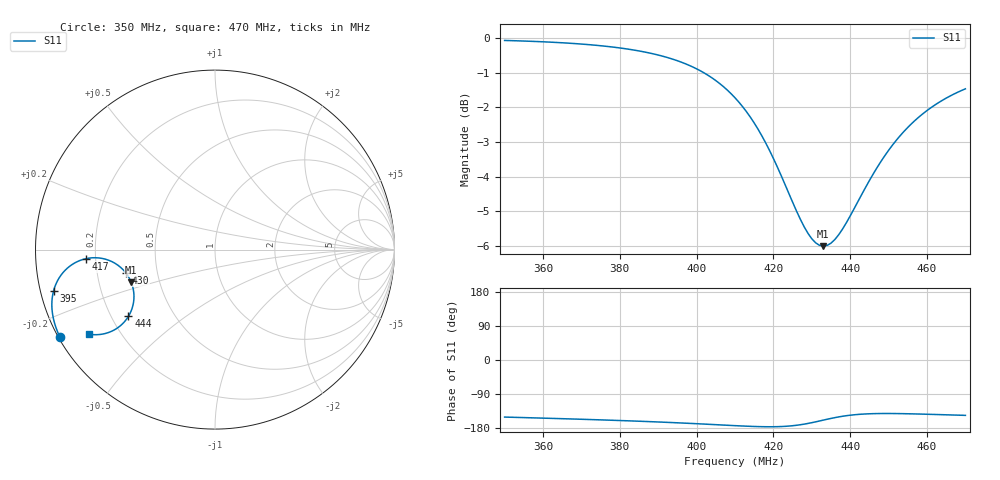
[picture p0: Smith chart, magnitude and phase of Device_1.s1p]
! Touchstone file exported from HFSS 2019.2.0
!  File:  C:/Users/Dana/Documents/Ansoft/New_Batwing_Rogers 5880_3.aedt
!  Generated:  2:31:46 PM  Apr 16, 2020
!  Design:  HFSSDesign1
!  Project:  New_Batwing_Rogers 5880_3
!  Setup:  Setup1
!  Solution:  Sweep
! Variables:
!  Bat_X = 12.5in
!  Bat_Y = 14.7in
!  Cavity_Spacing = 49.8mm
!  Cavity_X = 13.5in
!  Cavity_Y = 15in
!  Cavity_Z = 2in
!  Dog_Bone_Width = 10mm
!  Dog_Bone_length = 55mm
!  Feed_1_X = 1000009mm
!  Feed_1_X_extension = 999mm
!  Feed_2_Y = 2in
!  Feed_lower_Y = 24mm
!  Feed_lower_len = 65mm
!  Feed_lower_start = 15mm
!  Feed_upper_Y = 24mm
!  Feed_upper_leng = 999mm
!  Feed_upper_length = 20mm
!  Feed_upper_position = 8mm
!  Notch_X = 1.65in
!  Pin_X = 999
!  Pin_X_start_from_center = -2.475mm
!  Pin_diameter = 0.05in
!  Pin_inset = 2mm
!  Rad_Box_X = 392.9mm
!  Rad_Box_Y = 431mm
!  Rad_Box_Z = 90.8mm
!  Rad_Spacer = 215mm
!  Shorting_pin_diameter = 1.27mm
!  Slot_X = 10mm
!  Slot_Y = 14.16492in
!  Substrate_thickness = 0.062in
!  Tuner_length = 0mm
!  feed_1_X_start = 999
!  feed_1_Y = 999mm
!  feed_2_X = 999mm
!  rad_spacing = 9in
!  sf = 1
# GHZ S RI R 50.000000
! Modal data exported
! Port[1] = 1:1
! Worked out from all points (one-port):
!   121 points, 350 MHz to 470 MHz, reference 50 ohm
!   lowest |S11| = -6.0 dB at 433 MHz (marker M1), VSWR 3.01, Z = 17.2 - j8.36 ohm
!   |S11| at or under -10 dB: nowhere
!   S11 on the Smith chart (normalised r, x): 350 MHz: 0.00, -0.26; 395 MHz: 0.04, -0.12; 417 MHz: 0.16, -0.03; 430 MHz: 0.33, -0.11; 444 MHz: 0.27, -0.32; 470 MHz: 0.09, -0.30
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0.35  -0.8644 -0.4869
! Gamma ! 0 7.33545757681124
! Port Impedance50 0
0.365  -0.8913 -0.418
0.38  -0.9077 -0.3354
0.388  -0.908 -0.2822
0.395  -0.8989 -0.2285
0.399  -0.8873 -0.1947
0.403  -0.8691 -0.1591
0.407  -0.842 -0.1228
0.41  -0.8144 -0.0966
0.413  -0.7794 -0.0732
0.417  -0.7208 -0.0509
0.419  -0.6868 -0.0458
0.421  -0.6505 -0.0461
0.423  -0.6131 -0.0527
0.425  -0.576 -0.0662
0.427  -0.5411 -0.0868
0.43  -0.4968 -0.1295
0.433  -0.4665 -0.1826
0.436  -0.4525 -0.2398
0.438  -0.452 -0.2771
0.44  -0.4575 -0.3122
0.444  -0.4822 -0.3718
0.446  -0.499 -0.3956
0.449  -0.527 -0.424
0.452  -0.5561 -0.4446
0.455  -0.5848 -0.4587
0.462  -0.6453 -0.4733
0.47  -0.7013 -0.4712
